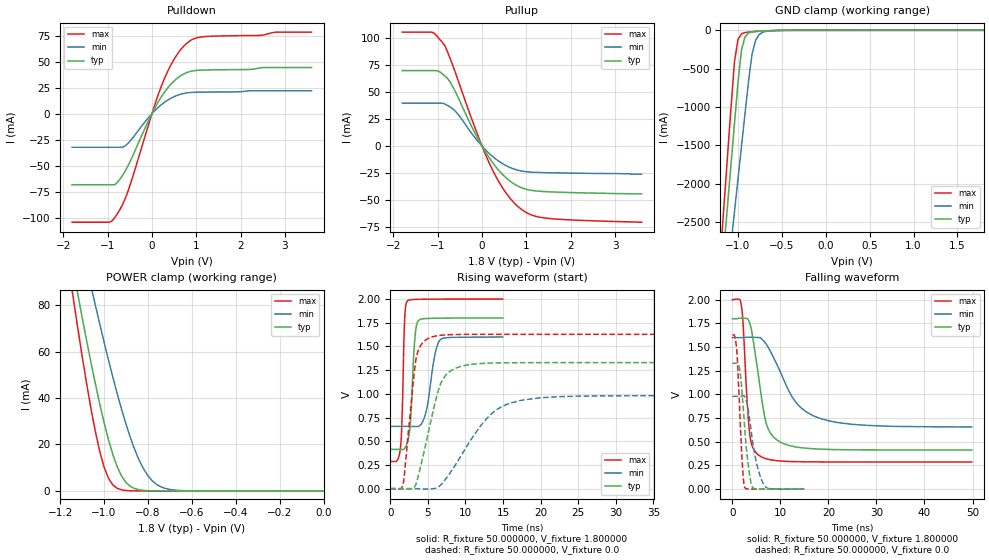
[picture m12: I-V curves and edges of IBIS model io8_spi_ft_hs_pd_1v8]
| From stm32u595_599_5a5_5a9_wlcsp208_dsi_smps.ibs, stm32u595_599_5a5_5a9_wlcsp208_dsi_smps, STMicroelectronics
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|   Model io8_spi_ft_hs_pd_1v8
[Model]  io8_spi_ft_hs_pd_1v8
Model_type I/O
Polarity   Non-Inverting
Enable   Active-Low
Vinl =   0.540000V
Vinh =   1.260000V
Vmeas =  0.900000V
Cref =   50.000000pF
Rref =   100.000000M
Vref =   0.0V
C_comp   3.338500pF   3.332300pF   3.378900pF
[Temperature Range]   25.000000   0.140000k   -40.000000
[Pullup Reference]   1.800000V   1.600000V   2.000000V
[Pulldown Reference]   0.0V   0.0V   0.0V
[POWER Clamp Reference]   1.800000V   1.600000V   2.000000V
[GND Clamp Reference]   0.0V   0.0V   0.0V
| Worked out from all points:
|   slope of the pulldown table from 0 to 0.27 V, typ, clamps not added: 13.6 ohm
|   slope of the pullup table from 0 to 0.27 V, typ, clamps not added: 15.9 ohm
|   GND clamp passes 1 mA (typ) near -0.50 V on its own axis
|   POWER clamp passes 1 mA (typ) near -0.86 V on its own axis
|   rising waveform, R_fixture 50.000000, V_fixture 1.800000: 20-80 % time 534ps typ, 1.08ns min, 336ps max; typ from 0.414 V to 1.8 V
|   rising waveform, R_fixture 50.000000, V_fixture 0.0: 20-80 % time 2.36ns typ, 5.18ns min, 1.21ns max; typ from 0 V to 1.33 V
|   falling waveform, R_fixture 50.000000, V_fixture 1.800000: 20-80 % time 2.6ns typ, 6.28ns min, 1.18ns max; typ from 1.8 V to 0.414 V
|   falling waveform, R_fixture 50.000000, V_fixture 0.0: 20-80 % time 1.33ns typ, 1.97ns min, 905ps max; typ from 1.33 V to 0 V
[Pulldown]
|Voltage   I(typ)   I(min)   I(max)
-1.8V     -68.38mA   -32.32mA   -104.4mA
-960mV    -68.38mA   -32.32mA   -104.4mA
-780mV    -66.07mA   -32.32mA   -96.42mA
-660mV    -59.2mA    -32.31mA   -87.22mA
-540mV    -50.22mA   -28.51mA   -74.66mA
0V        -10fA      -300fA     0A
240mV     18.04mA    9.599mA    29.41mA
480mV     30.68mA    16.02mA    50.95mA
780mV     39.47mA    19.98mA    67.56mA
960mV     41.44mA    20.62mA    72.37mA
1.14V     41.99mA    20.78mA    74.01mA
3.6V      44.44mA    22.06mA    78.55mA
[Pullup]
|Voltage   I(typ)   I(min)   I(max)
-1.8V     70.06mA    39.89mA    105.7mA
-1.14V    70.06mA    39.89mA    105.7mA
-1.02V    70.06mA    39.89mA    102.3mA
-840mV    65.11mA    39.14mA    93.15mA
-600mV    50.32mA    32.31mA    68.01mA
-180mV    13.77mA    8.913mA    19.32mA
180mV     -11.9mA    -7.442mA   -17.26mA
480mV     -26.98mA   -16.65mA   -39.76mA
840mV     -37.65mA   -22.63mA   -57.07mA
1.08V     -40.74mA   -24.01mA   -63.22mA
1.44V     -42.19mA   -24.58mA   -66.73mA
3.6V      -44.2mA    -26mA      -70.5mA
[GND_clamp]
|Voltage   I(typ)   I(min)   I(max)
-1.8V     -9.908A    -9.683A    -9.994A
-1.2V     -3.383A    -4.084A    -2.934A
-1.16V    -2.841A    -3.655A    -2.294A
-1.12V    -2.299A    -3.226A    -1.656A
-1.04V    -1.218A    -2.369A    -414.2mA
-1V       -684.7mA   -1.941A    -119.2mA
-960mV    -257.2mA   -1.514A    -45.67mA
-920mV    -87.04mA   -1.089A    -28.94mA
-840mV    -19.36mA   -312.8mA   -18.98mA
-800mV    -13.56mA   -132.4mA   -15.51mA
-720mV    -8.053mA   -25.67mA   -9.504mA
1.8V      45.71uA    33.32uA    56.11uA
[POWER_clamp]
|Voltage   I(typ)   I(min)   I(max)
-1.8V     470.8mA    433.7mA    554.6mA
-1.14V    95.25mA    122.7mA    82.82mA
-1.12V    84.97mA    114mA      70.27mA
-1.06V    55.51mA    88.42mA    35.67mA
-1.04V    46.34mA    80.15mA    25.76mA
-1V       29.51mA    64.13mA    10.3mA
-940mV    10.39mA    41.86mA    1.109mA
-900mV    3.624mA    28.77mA    182.8uA
-840mV    490.7uA    13.24mA    11.35uA
-800mV    116.8uA    6.532mA    1.77uA
-740mV    13.2uA     1.724mA    109.3nA
0V        0A         18.75nA    0A
[Ramp]
| variable   typ   min   max
dV/dt_r  0.79740/2.36103n   0.58782/5.17252n   0.97632/1.21227n
dV/dt_f  0.83141/2.59434n   0.56544/6.27737n   1.02743/1.18033n
R_load = 50.000000
[Rising Waveform]
R_fixture= 50.000000
V_fixture= 1.800000
V_fixture_min= 1.600000
V_fixture_max= 2.000000
|time   V(typ)   V(min)   V(max)
0s        413.8mV    656.5mV    287.1mV
1.351ns   413.1mV    656.5mV    427.6mV
1.562ns   412.1mV    656.5mV    736.1mV
1.892ns   422.5mV    656.5mV    1.747V
2.222ns   474mV      656.5mV    1.974V
2.673ns   691.3mV    656.3mV    1.992V
3.273ns   1.59V      654.9mV    1.995V
3.724ns   1.769V     656.2mV    1.996V
6.607ns   1.797V     1.567V     1.999V
14.95ns   1.8V       1.599V     1.999V
[Rising Waveform]
R_fixture= 50.000000
V_fixture= 0.0
V_fixture_min= 0.0
V_fixture_max= 0.0
|time   V(typ)   V(min)   V(max)
0s        1.365uV    2.257uV    4.637uV
1.702ns   -2.135mV   108.3nV    49.6mV
3.403ns   43.96mV    -269.1uV   1.358V
4.104ns   255.1mV    -3.342mV   1.517V
5.305ns   680.5mV    -3.257mV   1.593V
6.507ns   1.065V     23.36mV    1.615V
7.808ns   1.228V     149mV      1.623V
12.61ns   1.322V     719.7mV    1.627V
16.02ns   1.328V     902.8mV    1.627V
49.85ns   1.329V     979.8mV    1.627V
[Falling Waveform]
R_fixture= 50.000000
V_fixture= 1.800000
V_fixture_min= 1.600000
V_fixture_max= 2.000000
|time   V(typ)   V(min)   V(max)
0s        1.8V       1.599V     1.999V
1.902ns   1.805V     1.599V     1.927V
2.202ns   1.805V     1.599V     1.772V
3.604ns   1.754V     1.604V     586.2mV
5.606ns   1.132V     1.601V     354.4mV
6.907ns   723.8mV    1.54V      323.1mV
8.408ns   559.8mV    1.406V     306.7mV
12.71ns   450.7mV    953.3mV    290.9mV
17.02ns   426.2mV    770.7mV    287.9mV
49.85ns   413.8mV    656.5mV    287.1mV
[Falling Waveform]
R_fixture= 50.000000
V_fixture= 0.0
V_fixture_min= 0.0
V_fixture_max= 0.0
|time   V(typ)   V(min)   V(max)
0s        1.329V     979.8mV    1.627V
900.9ps   1.333V     979.8mV    1.475V
1.742ns   1.182V     980.4mV    585.2mV
2.252ns   867.2mV    985.5mV    134.6mV
2.613ns   610.7mV    974.1mV    14.87mV
3.273ns   268.7mV    846.1mV    2.532mV
4.054ns   36.88mV    561.9mV    1.21mV
5.075ns   2.952mV    266.2mV    716.6uV
6.486ns   1.088mV    53.26mV    415.3uV
14.95ns   1.365uV    2.257uV    4.637uV
